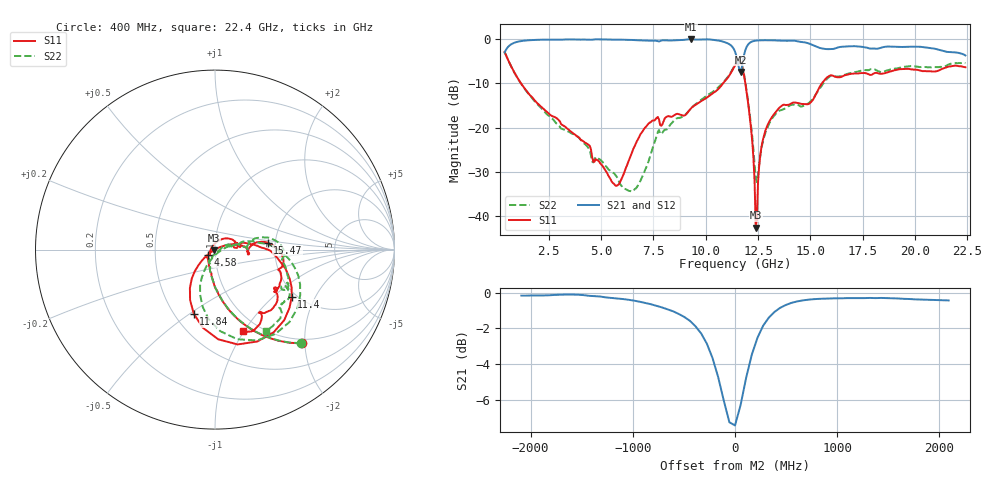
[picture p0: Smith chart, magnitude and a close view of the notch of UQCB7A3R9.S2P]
!  Part Number  UQCB7A3R9	Mounting Orientation: Vertical
!  Description: RF capacitors
!  Application: Coupling, Bypass, Tuning, DC Block
!  Filters, Matching
# GHZ S DB R 50
! Freq  |S11|  S11 Ph  |S21|  S21 Ph  |S12|  S12 Ph  |S22|  S22 Ph
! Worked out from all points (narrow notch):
!   401 points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, 400 MHz to 22.4 GHz, reference 50 ohm
!   highest |S21| = -0.04 dB at 9.31 GHz (marker M1); lowest = -7.4 dB at 11.68 GHz (marker M2)
!   notch at M2: 7.0 dB deep, 350 MHz wide at half that depth
!   lowest |S11| = -42.6 dB at 12.39 GHz (marker M3), VSWR 1.01, Z = 49.4 - j0.391 ohm
!   |S11| at or under -10 dB: 1.177 GHz to 10.83 GHz (9.657 GHz wide, 161 % of centre); 11.89 GHz to 15.55 GHz (3.661 GHz wide, 26.7 % of centre)
!   |S22| runs from -34.5 to -3.0 dB; largest |S21 - S12| = 0.0096
!   S11 on the Smith chart (normalised r, x): 400 MHz: 0.91, -1.93; 4.58 GHz: 0.93, -0.05; 11.4 GHz: 1.89, -1.32; 11.84 GHz: 0.62, -0.52; 15.47 GHz: 1.82, +0.15; 22.4 GHz: 0.83, -0.98
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0.4  -2.96 -47.3  -3.08 42.5  -3.10 42.5  -2.98 -47.3
0.84  -7.35 -70.1  -0.91 19.4  -0.93 19.5  -7.38 -70.1
1.39  -11.39 -83.5  -0.36 5.8  -0.38 5.8  -11.49 -83.6
4.085  -22.91 -121.2  -0.15 -24.6  -0.17 -24.6  -23.05 -118.9
4.58  -26.65 -143.0  -0.17 -28.4  -0.18 -28.3  -27.69 -123.1
5.735  -33.16 154.8  -0.16 -38.8  -0.19 -38.6  -30.98 -98.8
6.505  -25.28 68.3  -0.24 -45.3  -0.27 -45.0  -34.43 -41.3
7.77  -18.17 4.4  -0.59 -53.9  -0.54 -53.6  -20.57 9.7
9.31  -15.62 13.3  -0.04 -66.8  -0.01 -66.7  -15.61 15.9
10.74  -10.60 -0.1  -0.50 -85.1  -0.49 -85.1  -10.34 4.7
11.4  -6.00 -31.4  -2.86 -101.1  -2.85 -101.1  -5.82 -22.1
11.675  -5.30 -76.5  -7.44 -74.3  -7.42 -74.3  -5.07 -65.2
11.84  -8.48 -108.3  -3.46 -57.5  -3.45 -57.6  -8.19 -95.2
12.115  -18.02 -136.9  -0.85 -69.2  -0.83 -69.2  -17.43 -116.7
12.39  -42.60 -147.7  -0.39 -77.6  -0.37 -77.6  -31.47 -78.3
12.5  -32.26 27.3  -0.34 -80.0  -0.32 -80.0  -30.50 -14.9
12.72  -23.04 21.1  -0.31 -83.8  -0.29 -83.8  -23.40 11.9
13.105  -18.10 13.0  -0.29 -89.1  -0.28 -89.2  -18.49 13.7
15.085  -13.97 5.5  -1.32 -112.2  -1.31 -112.4  -13.70 13.1
15.47  -10.59 7.5  -2.07 -112.8  -2.03 -113.0  -11.06 14.1
18.77  -7.43 -35.5  -1.73 -128.6  -1.72 -128.6  -6.97 -27.9
22.4  -6.39 -71.3  -3.74 -164.4  -3.72 -164.8  -5.45 -57.9
